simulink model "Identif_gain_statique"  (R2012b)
settings: Solver=ode5  SolverMode=SingleTasking  StartTime=0.0  StopTime=inf  FixedStep=0.005  RelTol=1e-3  AbsTol=1e-6
undefined symbols (not defined in the file or in its folder): BaseAddress, T0

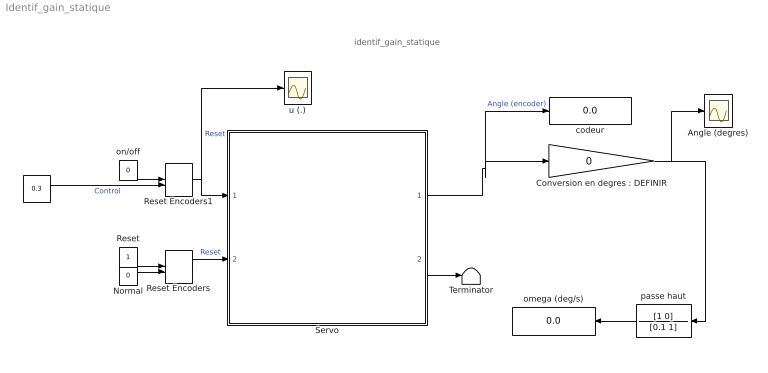
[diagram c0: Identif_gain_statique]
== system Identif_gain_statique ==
  note: identif_gain_statique
  " " : Constant  Value=0.3
  Angle (degres) : Scope
  "Conversion en degres : DEFINIR" : Gain  Gain=0
  Normal : Constant  Value=0
  Reset : Constant
  Reset Encoders : ManualSwitch  CurrentSetting=0
  Reset Encoders1 : ManualSwitch  CurrentSetting=0
  Servo : Subsystem
  Terminator : Terminator
  codeur : Display
  omega (deg/s) : Display
  on/off : Constant  Value=0
  passe haut : TransferFcn  Numerator=[1 0]  Denominator=[0.1 1]
  u (.) : Scope
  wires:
  Reset Encoders/1 -> Servo/2(Reset Encoder)  "Reset"
  Normal/1 -> Reset Encoders/2
  Reset/1 -> Reset Encoders/1
  "Conversion en degres : DEFINIR"/1 -> passe haut/1, Angle (degres)/1
  Servo/2(Set-up) -> Terminator/1
  Servo/1(Codeur_angulaire) -> codeur/1, "Conversion en degres : DEFINIR"/1  "Angle (encoder)"
  on/off/1 -> Reset Encoders1/1
  Reset Encoders1/1 -> u (.)/1, Servo/1(PWM Control)  "Reset"
  " "/1 -> Reset Encoders1/2  "Control"
  passe haut/1 -> omega (deg/s)/1

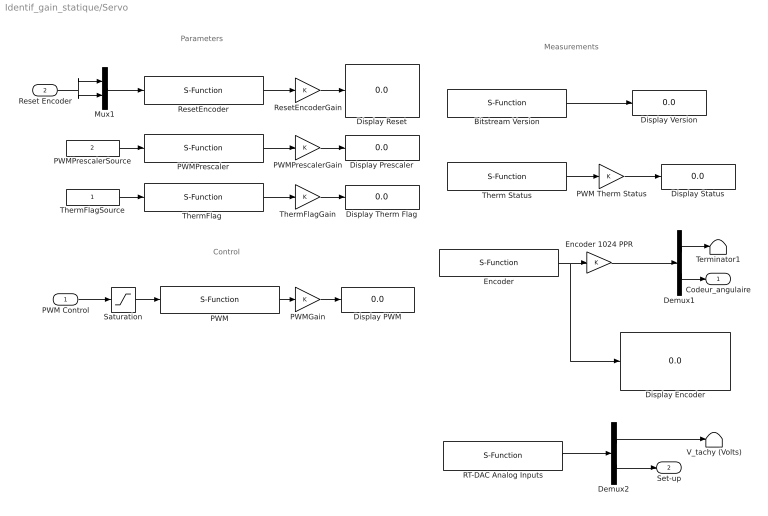
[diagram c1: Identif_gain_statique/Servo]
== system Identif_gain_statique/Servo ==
  note: Parameters
  note: Control
  note: Measurements
  PWM Control : Inport
  Reset Encoder : Inport  Port=2
  Bitstream Version : S-Function  FunctionName=Servo_BitstreamVersion  Parameters=BaseAddress, T0  EnableBusSupport=off
  Demux1 : Demux  Outputs=2
  Demux2 : Demux  Outputs=2
  Display Encoder : Display
  Display PWM : Display
  Display Prescaler : Display
  Display Reset : Display
  Display Status : Display
  Display Therm Flag : Display
  Display Version : Display
  Encoder : S-Function  FunctionName=Servo_Encoder  Parameters=BaseAddress, T0  EnableBusSupport=off
  Encoder 1024 PPR : Gain
  Mux1 : Mux  Inputs=2
  PWM : S-Function  FunctionName=Servo_PWM  Parameters=BaseAddress, T0  EnableBusSupport=off
  PWM Therm Status : Gain
  PWMGain : Gain
  PWMPrescaler : S-Function  FunctionName=Servo_PWMPrescaler  Parameters=BaseAddress, T0  EnableBusSupport=off
  PWMPrescalerGain : Gain
  PWMPrescalerSource : Constant  Value=2
  RT-DAC Analog Inputs : S-Function  FunctionName=servo_analoginputs  Parameters=BaseAddress, [1 0], [1 1], T0  EnableBusSupport=off
  ResetEncoder : S-Function  FunctionName=Servo_ResetEncoder  Parameters=BaseAddress, T0  EnableBusSupport=off
  ResetEncoderGain : Gain
  Saturation : Saturate  UpperLimit=1  LowerLimit=-1
  Terminator1 : Terminator
  Therm Status : S-Function  FunctionName=Servo_PWMTherm  Parameters=BaseAddress, T0  EnableBusSupport=off
  "ThermFlag " : S-Function  FunctionName=Servo_ThermFlag  Parameters=BaseAddress, T0  EnableBusSupport=off
  ThermFlagGain : Gain
  ThermFlagSource : Constant
  V_tachy (Volts) : Terminator
  Codeur_angulaire : Outport
  Set-up : Outport  Port=2
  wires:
  Encoder/1 -> Encoder 1024 PPR/1, Display Encoder/1
  Saturation/1 -> PWM/1
  PWM/1 -> PWMGain/1
  PWMGain/1 -> Display PWM/1
  ResetEncoder/1 -> ResetEncoderGain/1
  PWMPrescaler/1 -> PWMPrescalerGain/1
  Mux1/1 -> ResetEncoder/1
  PWMPrescalerSource/1 -> PWMPrescaler/1
  ResetEncoderGain/1 -> Display Reset/1
  PWMPrescalerGain/1 -> Display Prescaler/1
  PWM Control/1 -> Saturation/1
  Encoder 1024 PPR/1 -> Demux1/1
  Therm Status/1 -> PWM Therm Status/1
  PWM Therm Status/1 -> Display Status/1
  Bitstream Version/1 -> Display Version/1
  Reset Encoder/1 -> Mux1/1, Mux1/2
  "ThermFlag "/1 -> ThermFlagGain/1
  ThermFlagSource/1 -> "ThermFlag "/1
  ThermFlagGain/1 -> Display Therm Flag/1
  Demux1/1 -> Terminator1/1
  Demux1/2 -> Codeur_angulaire/1
  RT-DAC Analog Inputs/1 -> Demux2/1
  Demux2/2 -> Set-up/1
  Demux2/1 -> V_tachy (Volts)/1
